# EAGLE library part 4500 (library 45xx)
Industrial CONTROL UNIT
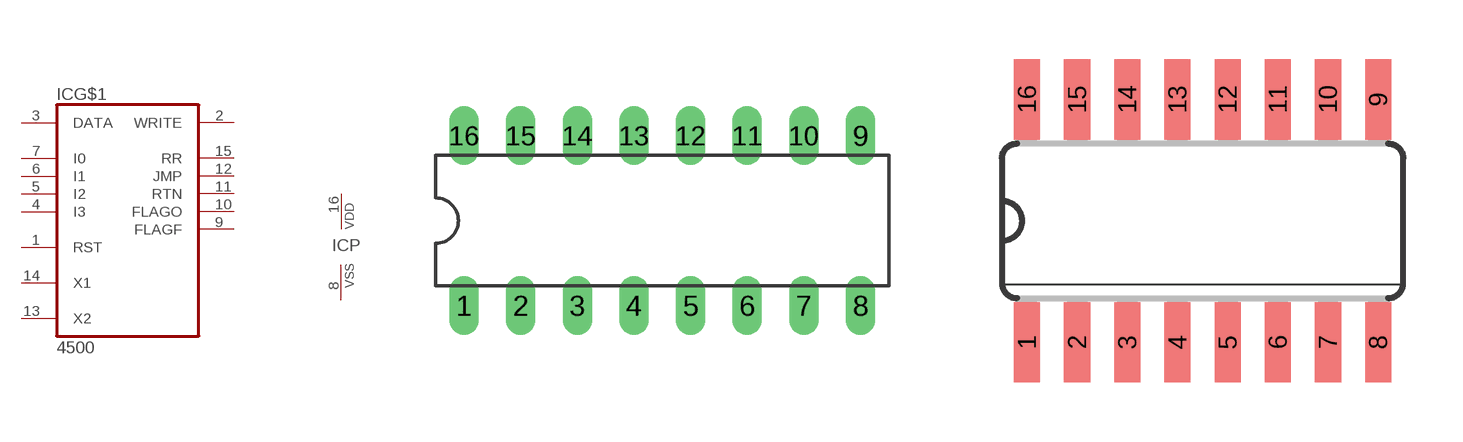
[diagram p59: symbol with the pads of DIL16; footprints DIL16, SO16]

Designator prefix IC; gates G$1=4500 P=PWRN

## 4500N  [DIL16]
1  G$1:RST  in
2  G$1:WRITE  out
3  G$1:DATA
4  G$1:I3  in
5  G$1:I2  in
6  G$1:I1  in
7  G$1:I0  in
8  P:VSS  pwr
9  G$1:FLAGF  out
10  G$1:FLAGO  out
11  G$1:RTN  out
12  G$1:JMP  out
13  G$1:X2  in
14  G$1:X1  out
15  G$1:RR  out
16  P:VDD  pwr

## 4500D  [SO16]
Pads as for DIL16

## Footprint DIL16 (pad centres in mm)
Dual In Line Package
drill 0.813 long: 1 -8.89,-3.81; 2 -6.35,-3.81; 3 -3.81,-3.81; 4 -1.27,-3.81; 5 1.27,-3.81; 6 3.81,-3.81; 7 6.35,-3.81; 8 8.89,-3.81; 9 8.89,3.81; 10 6.35,3.81; 11 3.81,3.81; 12 1.27,3.81; 13 -1.27,3.81; 14 -3.81,3.81; 15 -6.35,3.81; 16 -8.89,3.81

## Footprint SO16 (pad centres in mm)
Small Outline package 150 mil
smd 0.66 x 2.032: 1 -4.445,-3.073; 2 -3.175,-3.073; 3 -1.905,-3.073; 4 -0.635,-3.073; 5 0.635,-3.073; 6 1.905,-3.073; 7 3.175,-3.073; 8 4.445,-3.073; 9 4.445,3.073; 10 3.175,3.073; 11 1.905,3.073; 12 0.635,3.073; 13 -0.635,3.073; 14 -1.905,3.073; 15 -3.175,3.073; 16 -4.445,3.073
